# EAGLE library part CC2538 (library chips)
A Powerful System-On-Chip for 2.4-GHz IEEE 802.15.4, 6LoWPAN and ZigBee Applications
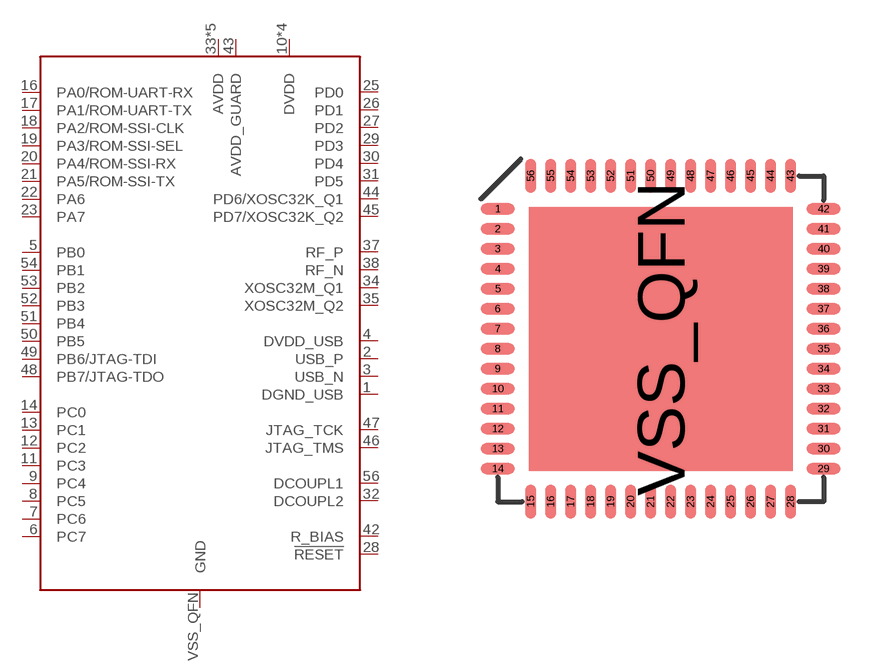
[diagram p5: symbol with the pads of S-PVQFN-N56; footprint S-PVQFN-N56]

Designator prefix U

## CC2538 (DIGIKEY: 296-35797-1-ND; MOUSER: 595-CC2538SF53RTQT; NEWARK: 87W7713)  [S-PVQFN-N56]
1  DGND_USB
2  USB_P
3  USB_N
4  DVDD_USB
5  PB0
6  PC7
7  PC6
8  PC5
9  PC4
10  DVDD
11  PC3
12  PC2
13  PC1
14  PC0
15  DVDD
16  PA0/ROM-UART-RX
17  PA1/ROM-UART-TX
18  PA2/ROM-SSI-CLK
19  PA3/ROM-SSI-SEL
20  PA4/ROM-SSI-RX
21  PA5/ROM-SSI-TX
22  PA6
23  PA7
24  DVDD
25  PD0
26  PD1
27  PD2
28  !RESET
29  PD3
30  PD4
31  PD5
32  DCOUPL2
33  AVDD
34  XOSC32M_Q1
35  XOSC32M_Q2
36  AVDD
37  RF_P
38  RF_N
39  AVDD
40  AVDD
41  AVDD
42  R_BIAS
43  AVDD_GUARD
44  PD6/XOSC32K_Q1
45  PD7/XOSC32K_Q2
46  JTAG_TMS
47  JTAG_TCK
48  PB7/JTAG-TDO
49  PB6/JTAG-TDI
50  PB5
51  PB4
52  PB3
53  PB2
54  PB1
55  DVDD
56  DCOUPL1
VSS_QFN  GND

## Footprint S-PVQFN-N56 (pad centres in mm)
S-PVQFN-N56
smd 0.85 x 0.28: 1 -4.075,3.25; 2 -4.075,2.75; 3 -4.075,2.25; 4 -4.075,1.75; 5 -4.075,1.25; 6 -4.075,0.75; 7 -4.075,0.25; 8 -4.075,-0.25; 9 -4.075,-0.75; 10 -4.075,-1.25; 11 -4.075,-1.75; 12 -4.075,-2.25; 13 -4.075,-2.75; 14 -4.075,-3.25; 29 4.075,-3.25; 30 4.075,-2.75; 31 4.075,-2.25; 32 4.075,-1.75; 33 4.075,-1.25; 34 4.075,-0.75; 35 4.075,-0.25; 36 4.075,0.25; 37 4.075,0.75; 38 4.075,1.25; 39 4.075,1.75; 40 4.075,2.25; 41 4.075,2.75; 42 4.075,3.25
smd 0.28 x 0.85: 15 -3.25,-4.075; 16 -2.75,-4.075; 17 -2.25,-4.075; 18 -1.75,-4.075; 19 -1.25,-4.075; 20 -0.75,-4.075; 21 -0.25,-4.075; 22 0.25,-4.075; 23 0.75,-4.075; 24 1.25,-4.075; 25 1.75,-4.075; 26 2.25,-4.075; 27 2.75,-4.075; 28 3.25,-4.075; 43 3.25,4.075; 44 2.75,4.075; 45 2.25,4.075; 46 1.75,4.075; 47 1.25,4.075; 48 0.75,4.075; 49 0.25,4.075; 50 -0.25,4.075; 51 -0.75,4.075; 52 -1.25,4.075; 53 -1.75,4.075; 54 -2.25,4.075; 55 -2.75,4.075; 56 -3.25,4.075
smd 6.6 x 6.6: VSS_QFN 0,0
